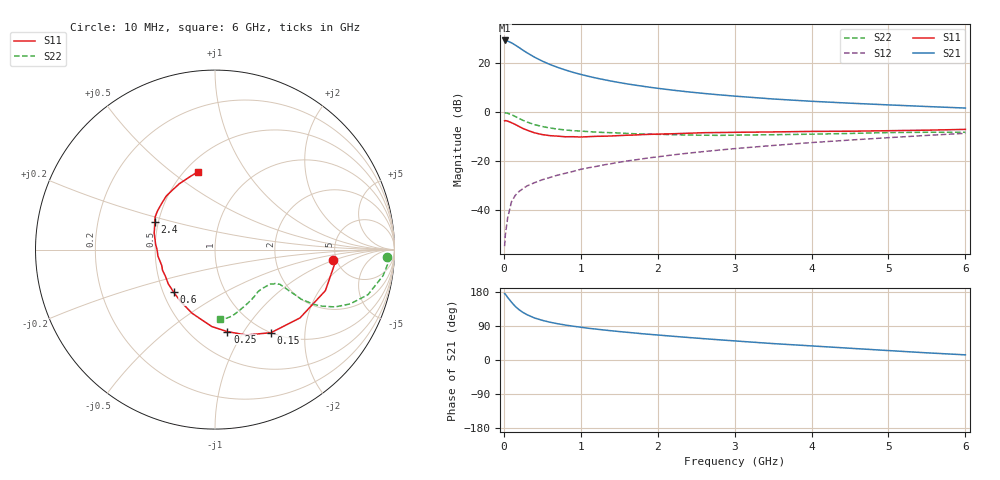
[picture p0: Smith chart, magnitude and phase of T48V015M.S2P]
! Infineon Technologies  Discrete & RF Semiconductors
! BFR182T
! Si NPN RF Bipolar Junction Transistor in SC75
! VCE = 8 V  IC = 15 mA
! Common Emitter S-Parameters:  October  1999
# GHz  S  MA  R  50
!  f  S11  S21  S12  S22
! GHz  MAG  ANG  MAG  ANG  MAG  ANG  MAG  ANG
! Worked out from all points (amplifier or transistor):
!   36 points, 10 MHz to 6 GHz, reference 50 ohm
!   highest |S21| = 29.4 dB at 10 MHz (marker M1)
!   |S21| within 3 dB of that: start of sweep to 202.5 MHz
!   unconditionally stable (mu >= 1): 880.5 MHz to 3.884 GHz
!   at 250 MHz: K = 0.53, MSG = 28.3 dB, |S12| = -31.3 dB
!   at 1.4 GHz: K = 1.07, MAG = 15.3 dB, |S12| = -21.1 dB
!   at 6 GHz: K = 0.87, MSG = 5.2 dB, |S12| = -8.7 dB
!   S11 on the Smith chart (normalised r, x): 10 MHz: 4.72, -0.97; 150 MHz: 1.00, -1.35; 250 MHz: 0.73, -0.85; 600 MHz: 0.57, -0.30; 2.4 GHz: 0.48, +0.17; 6 GHz: 0.58, +0.63
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0.01  0.6626 -5.0  29.43 175.3  0.0018 80.6  0.9612 -2.5
0.02  0.6716 -6.8  29.39 173.7  0.0031 89.5  0.9729 -3.5
0.05  0.6562 -20.4  28.55 165.1  0.0069 82.6  0.9477 -8.8
0.1  0.6075 -38.8  26.29 152.4  0.0147 74.0  0.8888 -16.4
0.15  0.5583 -56.0  23.62 141.1  0.0199 67.9  0.8116 -21.9
0.2  0.5069 -69.8  20.96 132.4  0.0239 65.6  0.7418 -25.5
0.25  0.4623 -81.4  18.53 125.4  0.0272 63.1  0.6787 -27.7
0.3  0.4289 -92.4  16.48 119.7  0.0308 62.1  0.6302 -29.0
0.4  0.3771 -109.8  13.35 110.8  0.036 61.1  0.5545 -29.9
0.5  0.3471 -123.5  11.11 104.7  0.0413 62.2  0.5077 -29.4
0.6  0.3303 -134.4  9.466 99.7  0.046 63.7  0.4744 -29.1
0.8  0.3136 -151.8  7.312 92.2  0.056 65.2  0.4321 -28.4
0.9  0.3142 -158.6  6.54 89.2  0.0611 66.1  0.4175 -28.3
1.1  0.315 -169.9  5.427 83.7  0.0726 67.0  0.3994 -28.7
1.3  0.3217 -178.5  4.639 79.2  0.0833 67.5  0.3835 -29.5
1.6  0.3368 171.6  3.802 73.1  0.1001 67.7  0.3668 -31.4
2.2  0.3616 158.5  2.82 62.6  0.1334 67.3  0.3462 -37.4
2.4  0.37 155.0  2.601 59.4  0.1448 67.1  0.3398 -39.8
3.5  0.3937 138.5  1.862 43.3  0.2079 63.1  0.3455 -54.1
4.5  0.4073 126.1  1.528 31.0  0.2684 58.3  0.3666 -68.6
5.5  0.4279 109.9  1.305 18.9  0.3342 52.8  0.3877 -80.6
6  0.4439 102.3  1.214 13.6  0.3688 49.3  0.3885 -85.5
